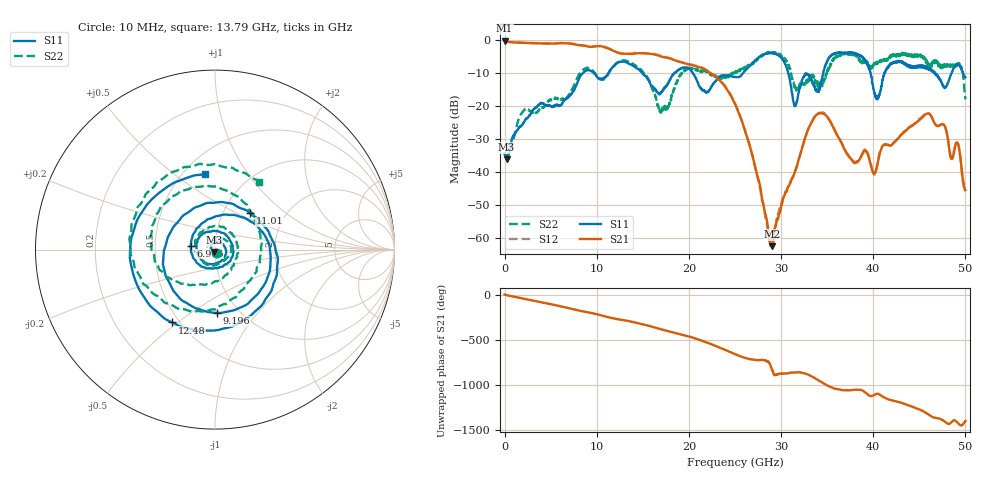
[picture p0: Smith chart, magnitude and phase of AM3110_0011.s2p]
# Hz S DB R 50.0
!freq dBS11 angS11 dBS21 angS21 dBS12 angS12 dBS22 angS22
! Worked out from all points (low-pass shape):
!   1601 points, 10 MHz to 50 GHz, reference 50 ohm
!   highest |S21| = -0.12 dB at 10 MHz (marker M1); lowest = -62.5 dB at 29 GHz (marker M2)
!   |S21| within 3 dB of the highest: start of sweep to 11.78 GHz
!   lowest |S11| = -36.2 dB at 228.7 MHz (marker M3), VSWR 1.03, Z = 49.4 - j1.42 ohm
!   |S11| at or under -10 dB: start of sweep to 8.488 GHz; 20.43 GHz to 25.86 GHz (5.437 GHz wide, 23.5 % of centre); 30.78 GHz to 34.58 GHz (3.8 GHz wide, 11.6 % of centre)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
!   |S22| runs from -35.3 to -3.5 dB; largest |S21 - S12| = 0.021
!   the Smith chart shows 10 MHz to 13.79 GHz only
!   S11 on the Smith chart (normalised r, x): 10 MHz: 1.01, -0.04; 6.915 GHz: 0.76, +0.03; 9.196 GHz: 0.79, -0.64; 11.01 GHz: 1.33, +0.59; 12.48 GHz: 0.46, -0.48; 13.79 GHz: 0.64, +0.65
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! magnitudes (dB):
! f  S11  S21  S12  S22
! 10 MHz  -34.7  -0.1  0.0  -33.9
! 228.7 MHz  -36.2  -0.3  -0.2  -35.2
! 2.103 GHz  -24.8  -0.8  -0.7  -21.2
! 6.915 GHz  -17.2  -0.9  -0.8  -16.8
! 8.352 GHz  -10.3  -1.5  -1.5  -9.3
! 9.196 GHz  -9.0  -1.9  -1.7  -8.4
! 11.01 GHz  -11.0  -2.2  -2.0  -11.3
! 12.48 GHz  -6.6  -3.9  -3.9  -6.4
! 13.79 GHz  -7.5  -4.1  -3.9  -7.0
! 16.69 GHz  -16.1  -4.6  -4.4  -20.0
! 19.82 GHz  -8.4  -7.2  -7.1  -8.5
! 21.88 GHz  -15.9  -9.1  -8.9  -9.2
! 25 GHz  -11.1  -19.3  -19.1  -9.8
! 29 GHz  -3.9  -62.5  -60.7  -3.7
! 31.5 GHz  -19.9  -39.8  -40.2  -14.7
! 33.35 GHz  -12.1  -24.8  -24.5  -10.2
! 37.75 GHz  -3.7  -36.6  -36.5  -4.1
! 40.1 GHz  -15.6  -40.6  -40.2  -6.9
! 41.69 GHz  -7.8  -31.8  -31.6  -5.8
! 46.06 GHz  -8.9  -22.3  -22.1  -7.3
! 49.16 GHz  -7.2  -31.3  -31.0  -7.6
! 50 GHz  -11.2  -45.5  -45.4  -17.9
